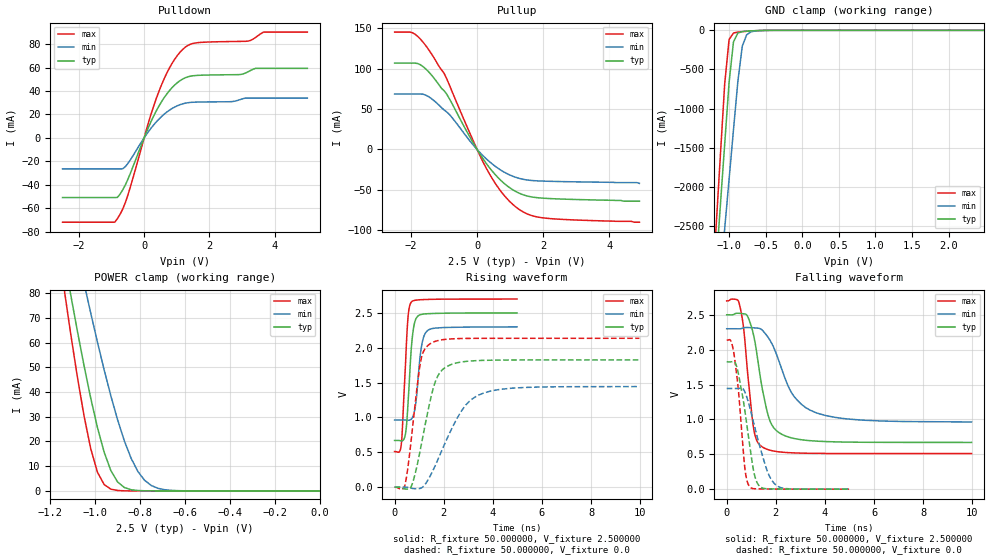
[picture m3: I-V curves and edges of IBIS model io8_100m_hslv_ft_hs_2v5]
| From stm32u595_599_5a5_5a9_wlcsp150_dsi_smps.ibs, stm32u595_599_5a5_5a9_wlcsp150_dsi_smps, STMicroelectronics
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|   Model io8_100m_hslv_ft_hs_2v5
[Model]  io8_100m_hslv_ft_hs_2v5
Model_type I/O
Polarity   Non-Inverting
Enable   Active-Low
Vinl =   0.750000V
Vinh =   1.750000V
Vmeas =  1.250000V
Cref =   50.000000pF
Rref =   100.000000M
Vref =   0.0V
C_comp   3.340900pF   3.338500pF   3.380300pF
[Temperature Range]   25.000000   0.140000k   -40.000000
[Pullup Reference]   2.500000V   2.300000V   2.700000V
[Pulldown Reference]   0.0V   0.0V   0.0V
[POWER Clamp Reference]   2.500000V   2.300000V   2.700000V
[GND Clamp Reference]   0.0V   0.0V   0.0V
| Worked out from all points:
|   slope of the pulldown table from 0 to 0.375 V, typ, clamps not added: 16.1 ohm
|   slope of the pullup table from 0 to 0.375 V, typ, clamps not added: 16.6 ohm
|   GND clamp passes 1 mA (typ) near -0.50 V on its own axis
|   POWER clamp passes 1 mA (typ) near -0.86 V on its own axis
|   rising waveform, R_fixture 50.000000, V_fixture 2.500000: 20-80 % time 200ps typ, 231ps min, 180ps max; typ from 0.67 V to 2.5 V
|   rising waveform, R_fixture 50.000000, V_fixture 0.0: 20-80 % time 660ps typ, 1.22ns min, 424ps max; typ from 0 V to 1.82 V
|   falling waveform, R_fixture 50.000000, V_fixture 2.500000: 20-80 % time 569ps typ, 1.09ns min, 362ps max; typ from 2.5 V to 0.67 V
|   falling waveform, R_fixture 50.000000, V_fixture 0.0: 20-80 % time 467ps typ, 672ps min, 321ps max; typ from 1.82 V to 0 V
[Pulldown]
|Voltage   I(typ)   I(min)   I(max)
-2.5V     -51mA      -26.45mA   -72.04mA
-900mV    -51mA      -26.45mA   -72.04mA
-820mV    -50.89mA   -26.45mA   -69.09mA
-500mV    -35.59mA   -21.93mA   -49.09mA
140mV     9.489mA    5.639mA    13.76mA
460mV     27.5mA     16.24mA    40.22mA
860mV     43.07mA    25.18mA    63.88mA
1.26V     51.38mA    29.65mA    77.49mA
1.66V     53.45mA    30.63mA    81.42mA
3.18V     56.44mA    34.01mA    82.68mA
3.66V     59.44mA    34.01mA    90.42mA
5V        59.44mA    34.01mA    90.42mA
[Pullup]
|Voltage   I(typ)   I(min)   I(max)
-2.5V     106.8mA    68.58mA    145.2mA
-1.96V    106.8mA    68.58mA    144.4mA
-1.72V    104.8mA    68.58mA    136.6mA
-1.48V    96.52mA    65.55mA    124.2mA
-1V       72.68mA    48.88mA    94.23mA
-120mV    8.307mA    5.657mA    10.97mA
280mV     -17.4mA    -11.68mA   -23.32mA
680mV     -36.72mA   -24.56mA   -49.54mA
1.16V     -51.75mA   -34.32mA   -70.71mA
1.56V     -58mA      -38.01mA   -80.45mA
1.96V     -60.18mA   -39.11mA   -84.44mA
4.92V     -64mA      -42mA      -90mA
[GND_clamp]
|Voltage   I(typ)   I(min)   I(max)
-2.5V     -9.446A    -9.524A    -9.146A
-1.18V    -3.045A    -3.8A      -2.552A
-1.12V    -2.248A    -3.166A    -1.614A
-1.06V    -1.452A    -2.533A    -685.3mA
-1V       -665mA     -1.901A    -117.9mA
-940mV    -148mA     -1.272A    -34.32mA
-880mV    -35.13mA   -651.5mA   -22.79mA
-820mV    -16mA      -203.9mA   -17.07mA
-760mV    -10.46mA   -56.88mA   -12.26mA
-700mV    -7.068mA   -18.52mA   -8.146mA
-400mV    -103.3uA   -375.9uA   -42.12uA
2.48V     0A         14.84nA    0A
[POWER_clamp]
|Voltage   I(typ)   I(min)   I(max)
-2.49V    881mA      773.1mA    1.07A
-1.14V    95.25mA    122.7mA    82.82mA
-1.11V    79.9mA     109.7mA    64.14mA
-1.05V    50.87mA    84.26mA    30.57mA
-1.02V    37.63mA    72.04mA    17.17mA
-990mV    25.71mA    60.25mA    7.621mA
-930mV    8.217mA    38.43mA    713.9uA
-900mV    3.624mA    28.77mA    182.8uA
-840mV    490.7uA    13.24mA    11.35uA
-780mV    56.55uA    4.324mA    699nA
-660mV    716.5nA    226uA      9.775nA
0V        0A         19.49nA    0A
[Ramp]
| variable   typ   min   max
dV/dt_r  1.09506/0.65941n   0.86580/1.21842n   1.28196/0.42320n
dV/dt_f  1.09807/0.56793n   0.80135/1.08586n   1.31359/0.36130n
R_load = 50.000000
[Rising Waveform]
R_fixture= 50.000000
V_fixture= 2.500000
V_fixture_min= 2.300000
V_fixture_max= 2.700000
|time   V(typ)   V(min)   V(max)
0s        670mV      963.2mV    510.4mV
270.3ps   664.3mV    963.5mV    606.4mV
450.5ps   780.3mV    962.9mV    1.815V
550.6ps   1.224V     960mV      2.454V
680.7ps   1.993V     976.4mV    2.655V
760.8ps   2.258V     1.028V     2.675V
870.9ps   2.417V     1.23V      2.684V
1.081ns   2.478V     1.989V     2.69V
1.341ns   2.489V     2.247V     2.694V
4.985ns   2.5V       2.3V       2.699V
[Rising Waveform]
R_fixture= 50.000000
V_fixture= 0.0
V_fixture_min= 0.0
V_fixture_max= 0.0
|time   V(typ)   V(min)   V(max)
0s        -146.1uV   -65.64uV   -358.8uV
400.4ps   -24.12mV   -179.4uV   3.555mV
680.7ps   11.58mV    -15.32mV   692.2mV
1.081ns   598mV      -13.77mV   1.838V
1.461ns   1.258V     168.7mV    2.06V
1.702ns   1.551V     346.1mV    2.097V
2.002ns   1.701V     590mV      2.118V
2.723ns   1.796V     1.092V     2.133V
3.423ns   1.817V     1.321V     2.135V
9.97ns    1.825V     1.443V     2.136V
[Falling Waveform]
R_fixture= 50.000000
V_fixture= 2.500000
V_fixture_min= 2.300000
V_fixture_max= 2.700000
|time   V(typ)   V(min)   V(max)
0s        2.5V       2.3V       2.699V
520.5ps   2.521V     2.299V     2.648V
700.7ps   2.514V     2.314V     2.272V
1.101ns   2.2V       2.313V     862.5mV
1.461ns   1.418V     2.275V     602.6mV
1.722ns   1.019V     2.158V     562.4mV
1.962ns   861.5mV    1.993V     543.2mV
2.623ns   736.7mV    1.395V     521.4mV
3.403ns   694.8mV    1.131V     513.9mV
9.97ns    670mV      963.2mV    510.4mV
[Falling Waveform]
R_fixture= 50.000000
V_fixture= 0.0
V_fixture_min= 0.0
V_fixture_max= 0.0
|time   V(typ)   V(min)   V(max)
0s        1.825V     1.443V     2.136V
300.3ps   1.831V     1.443V     1.932V
470.5ps   1.666V     1.444V     1.443V
740.7ps   1.124V     1.394V     300.7mV
930.9ps   645mV      1.183V     36.36mV
1.121ns   222.8mV    919mV      6.541mV
1.281ns   66.87mV    699.5mV    4.001mV
1.662ns   5.708mV    251.8mV    2.109mV
2.002ns   3.185mV    60.93mV    1.18mV
4.985ns   -146.1uV   -65.64uV   -358.8uV
